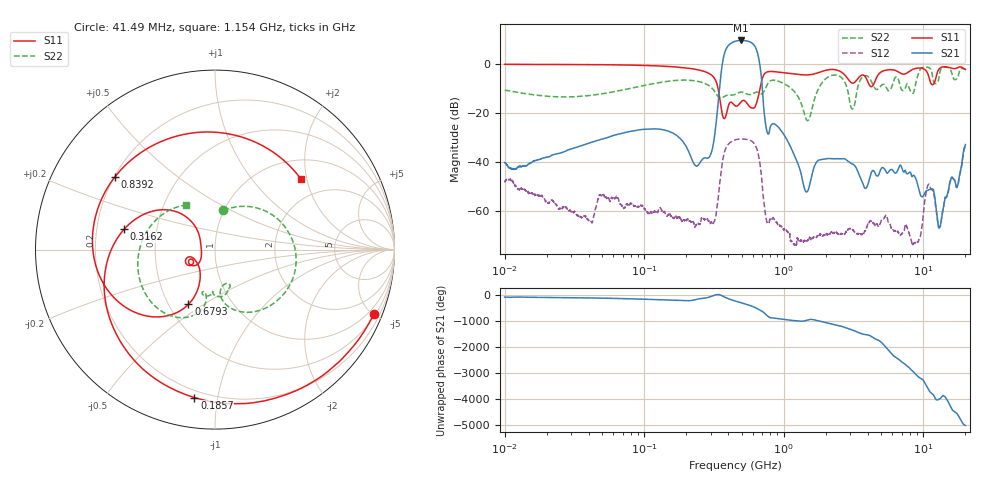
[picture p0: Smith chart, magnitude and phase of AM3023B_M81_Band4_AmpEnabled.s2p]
!Agilent Technologies,E8364B,MY43040894,A.07.50.67
!Agilent E8364B: A.07.50.67
!Date: Tuesday, October 27, 2020 10:43:40
!Correction: S11(Full 2 Port(1,2))
!S21(Full 2 Port(1,2))
!S12(Full 2 Port(1,2))
!S22(Full 2 Port(1,2))
!S2P File: Measurements: S11, S21, S12, S22:Log Frequency Sweep
# Hz S  dB  R 50
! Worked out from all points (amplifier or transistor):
!   3201 points, 10 MHz to 20 GHz, reference 50 ohm
!   highest |S21| = 9.4 dB at 494.1 MHz (marker M1)
!   |S21| within 3 dB of that: 390.3 MHz to 629.1 MHz (238.8 MHz wide, 46.9 % of centre)
!   unconditionally stable (mu >= 1): start of sweep to end of sweep
!   at 35.47 MHz: K = 2650.69, MAG = -22.7 dB, |S12| = -62.5 dB
!   at 447.2 MHz: K = 5.82, MAG = 9.4 dB, |S12| = -31.0 dB
!   at 20 GHz: K = 182.44, MAG = -25.4 dB, |S12| = -33.4 dB
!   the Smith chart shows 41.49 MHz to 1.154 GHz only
!   S11 on the Smith chart (normalised r, x): 41.49 MHz: 0.63, -5.07; 185.7 MHz: 0.16, -0.86; 316.2 MHz: 0.32, +0.10; 679.3 MHz: 0.63, -0.43; 839.2 MHz: 0.20, +0.31; 1.154 GHz: 1.44, +1.84
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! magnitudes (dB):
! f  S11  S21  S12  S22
! 10 MHz  -0.3  -40.2  -47.7  -10.8
! 35.55 MHz  -0.4  -33.4  -62.6  -13.3
! 41.49 MHz  -0.4  -32.1  -64.2  -12.9
! 126.1 MHz  -1.0  -26.6  -59.8  -7.8
! 185.7 MHz  -1.6  -31.1  -64.3  -6.7
! 237.7 MHz  -2.4  -41.8  -65.4  -7.1
! 316.2 MHz  -5.7  -31.1  -64.4  -10.9
! 371.6 MHz  -22.3  3.0  -37.1  -13.5
! 447.2 MHz  -17.1  9.1  -31.0  -12.5
! 494.1 MHz  -15.5  9.4  -30.7  -11.6
! 679.3 MHz  -9.4  -2.0  -41.8  -12.2
! 754.2 MHz  -3.5  -27.1  -64.3  -9.0
! 839.2 MHz  -3.2  -24.5  -63.0  -6.7
! 1.154 GHz  -4.2  -35.6  -72.7  -10.6
! 1.59 GHz  -4.4  -45.2  -71.5  -18.5
! 2.212 GHz  -2.4  -38.7  -68.6  -4.8
! 3.099 GHz  -7.9  -40.9  -67.5  -18.4
! 5.639 GHz  -2.5  -44.0  -64.5  -11.1
! 8.94 GHz  -1.9  -47.7  -72.6  -6.5
! 11.02 GHz  -6.0  -51.2  -49.1  -1.7
! 13.07 GHz  -2.0  -66.7  -66.5  -4.0
! 20 GHz  -2.4  -32.9  -33.4  -2.3
